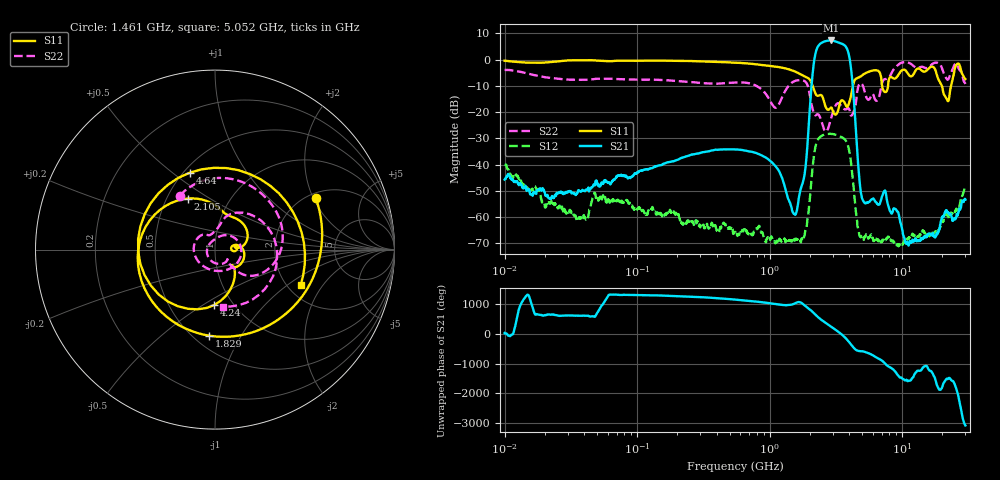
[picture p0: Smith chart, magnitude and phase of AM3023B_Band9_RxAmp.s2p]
# Hz S DB R 50.0
!freq dBS11 angS11 dBS21 angS21 dBS12 angS12 dBS22 angS22
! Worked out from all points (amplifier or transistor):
!   1601 points, 10 MHz to 30 GHz, reference 50 ohm
!   highest |S21| = 7.3 dB at 2.899 GHz (marker M1)
!   |S21| within 3 dB of that: 2.278 GHz to 3.821 GHz (1.543 GHz wide, 50.6 % of centre)
!   unconditionally stable (mu >= 1): start of sweep to end of sweep
!   at 37.85 MHz: K = 6282.78, MAG = -36.0 dB, |S12| = -60.4 dB
!   at 547.7 MHz: K = 10177.33, MAG = -27.4 dB, |S12| = -65.6 dB
!   at 30 GHz: K = 41226.24, MAG = -52.0 dB, |S12| = -47.8 dB
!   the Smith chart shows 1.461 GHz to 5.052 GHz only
!   S11 on the Smith chart (normalised r, x): 1.461 GHz: 2.19, +2.09; 1.829 GHz: 0.59, -0.74; 2.105 GHz: 0.64, +0.40; 4.24 GHz: 0.82, -0.56; 4.64 GHz: 0.54, +0.58; 5.052 GHz: 2.35, -1.27
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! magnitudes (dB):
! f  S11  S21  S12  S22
! 10 MHz  -0.4  -45.7  -40.1  -3.9
! 38.04 MHz  -0.2  -50.0  -60.7  -7.7
! 48.37 MHz  -0.3  -46.6  -51.1  -7.3
! 144.7 MHz  -0.4  -40.3  -58.6  -7.7
! 547.7 MHz  -1.2  -34.2  -65.6  -8.7
! 1.06 GHz  -2.5  -39.6  -68.8  -17.5
! 1.461 GHz  -4.0  -56.4  -69.2  -8.9
! 1.829 GHz  -6.4  -44.2  -67.3  -8.1
! 2.084 GHz  -9.2  -8.3  -44.0  -17.7
! 2.105 GHz  -9.8  -5.9  -41.5  -18.6
! 2.314 GHz  -13.8  5.0  -30.4  -20.8
! 2.899 GHz  -18.3  7.3  -28.3  -22.6
! 3.798 GHz  -17.8  4.6  -31.3  -18.8
! 4.24 GHz  -10.2  -10.1  -45.5  -20.6
! 4.64 GHz  -6.9  -39.0  -64.3  -10.7
! 5.052 GHz  -5.7  -53.6  -68.0  -9.9
! 7.926 GHz  -7.7  -56.3  -67.5  -6.7
! 10.92 GHz  -4.9  -69.6  -68.6  -1.0
! 17.04 GHz  -2.7  -66.3  -66.0  -1.5
! 21.78 GHz  -15.2  -57.7  -59.2  -7.4
! 25.95 GHz  -1.7  -58.9  -57.0  -1.6
! 30 GHz  -7.4  -53.4  -47.8  -9.2
